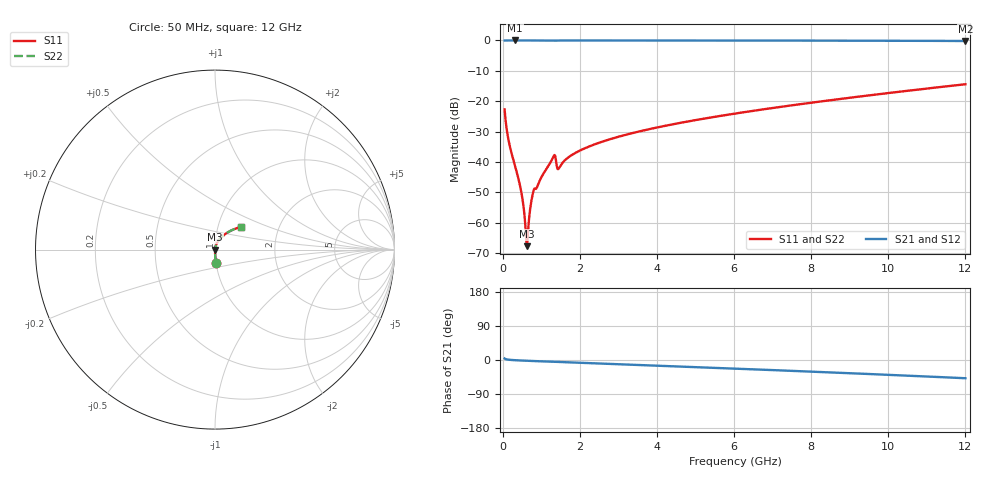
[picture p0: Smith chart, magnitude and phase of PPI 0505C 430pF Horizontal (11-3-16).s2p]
# MHz S MA R 50
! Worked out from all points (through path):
!   1601 points, 50 MHz to 12 GHz, reference 50 ohm
!   highest |S21| = 0.00 dB at 318.9 MHz (marker M1); lowest = -0.2 dB at 12 GHz (marker M2)
!   group delay of S21, straight-line fit = 11.1 ps
!   lowest |S11| = -67.7 dB at 625.1 MHz (marker M3), VSWR 1.00, Z = 50 - j0.00655 ohm
!   |S11| at or under -10 dB: start of sweep to end of sweep
!   |S22| runs from -67.7 to -14.4 dB; largest |S21 - S12| = 0
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50  0.07327 -85.8  0.9971 4.0  0.9971 4.0  0.07327 -85.8
169.5  0.02025 -88.7  0.9995 0.6  0.9995 0.6  0.02025 -88.7
318.875  0.008669 -88.5  0.9996 -0.5  0.9996 -0.5  0.008669 -88.5
475.7188  0.00339 -85.2  0.9996 -1.3  0.9996 -1.3  0.00339 -85.2
528  0.002133 -81.5  0.9996 -1.6  0.9996 -1.6  0.002133 -81.5
587.75  0.0008943 -65.7  0.9996 -1.8  0.9996 -1.8  0.0008943 -65.7
625.0938  0.0004124 -9.1  0.9996 -2.0  0.9996 -2.0  0.0004124 -9.1
662.4375  0.0007956 55.2  0.9995 -2.2  0.9995 -2.2  0.0007956 55.2
737.125  0.00214 73.5  0.9994 -2.5  0.9994 -2.5  0.00214 73.5
767  0.002719 74.2  0.9993 -2.6  0.9993 -2.6  0.002719 74.2
804.3438  0.003433 71.3  0.999 -2.8  0.999 -2.8  0.003433 71.3
1297.281  0.01162 74.4  0.9977 -4.8  0.9977 -4.8  0.01162 74.4
1342.094  0.01305 62.4  0.9948 -5.0  0.9948 -5.0  0.01305 62.4
1461.594  0.007973 69.6  0.9978 -5.1  0.9978 -5.1  0.007973 69.6
1693.125  0.01179 80.0  0.999 -6.1  0.999 -6.1  0.01179 80.0
2044.156  0.01588 80.0  0.999 -7.5  0.999 -7.5  0.01588 80.0
2865.719  0.02458 77.7  0.9988 -10.6  0.9988 -10.6  0.02458 77.7
4038.312  0.03739 73.7  0.9982 -15.1  0.9982 -15.1  0.03739 73.7
6025  0.06263 66.4  0.9967 -22.7  0.9967 -22.7  0.06263 66.4
8019.156  0.09486 58.6  0.9938 -30.8  0.9938 -30.8  0.09486 58.6
10013.31  0.1366 50.3  0.9886 -39.2  0.9886 -39.2  0.1366 50.3
12000  0.1901 41.4  0.9794 -48.1  0.9794 -48.1  0.1901 41.4
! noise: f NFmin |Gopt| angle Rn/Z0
50  0.0003043  0.8298  0.2344  0.0003767
1372  0.00974  0.8525  4.403  0.01406
2701  0.004629  0.5047  8.348  0.001611
4031  0.006124  0.4602  12.21  0.001889
5360  0.007565  0.433  15.94  0.002166
6682  0.008974  0.4157  19.49  0.002444
8012  0.0104  0.4052  22.89  0.002737
9341  0.01186  0.4004  26.15  0.003055
1.067e+04  0.01338  0.4004  29.26  0.003411
1.2e+04  0.01499  0.4048  32.25  0.003816
